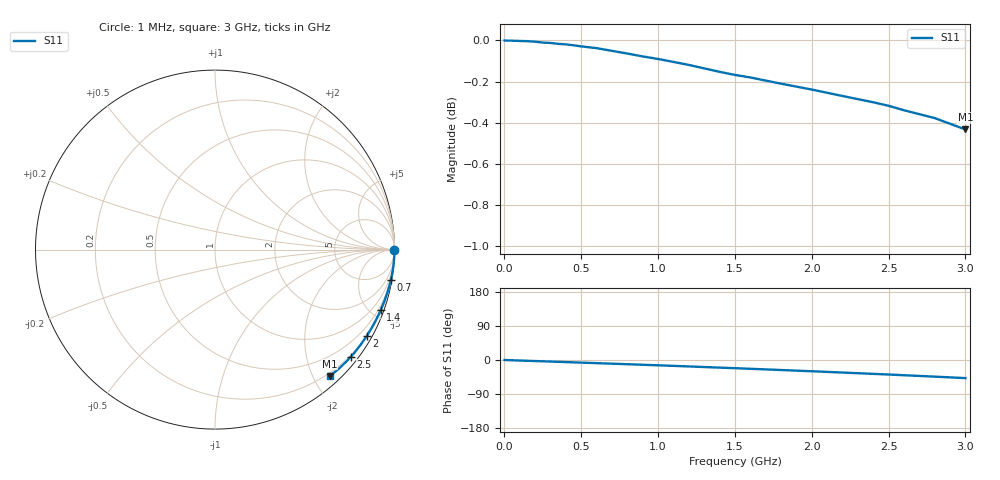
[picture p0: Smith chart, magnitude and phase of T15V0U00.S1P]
! SIEMENS Small Signal Semiconductors
! BAT68-04
! Si Schottky Diode (2 diodes in series, pin 3 open) in SOT23
! VR = 5 V
! S-Parameters:  August  1994
# GHz  S  MA  R  50
!  f  S11
! GHz  MAG  ANG
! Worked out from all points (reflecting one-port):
!   33 points, 1 MHz to 3 GHz, reference 50 ohm
!   lowest |S11| = -0.4 dB at 3 GHz (marker M1), VSWR 40.15, Z = 7.56 - j112 ohm
!   phase of S11 starts at 0 deg and turns -48 deg over the sweep
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0.001  1 0.0
0.003  1 0.0
0.05  0.9999 -0.7
0.06  0.9998 -0.8
0.1  0.9997 -1.4
0.15  0.9996 -2.1
0.2  0.9993 -2.8
0.25  0.9988 -3.4
0.3  0.9986 -4.1
0.4  0.9978 -5.5
0.45  0.9973 -6.2
0.6  0.9957 -8.3
0.7  0.9942 -9.7
0.8  0.9927 -11.1
0.9  0.9911 -12.6
1  0.9897 -14.0
1.2  0.9864 -17.0
1.4  0.9826 -20.1
1.5  0.9809 -21.6
1.6  0.9795 -23.2
1.8  0.9761 -26.4
2  0.9729 -29.7
2.2  0.9694 -33.1
2.4  0.966 -36.6
2.5  0.9641 -38.3
2.6  0.9617 -40.2
2.8  0.9575 -43.9
3  0.9514 -47.8
